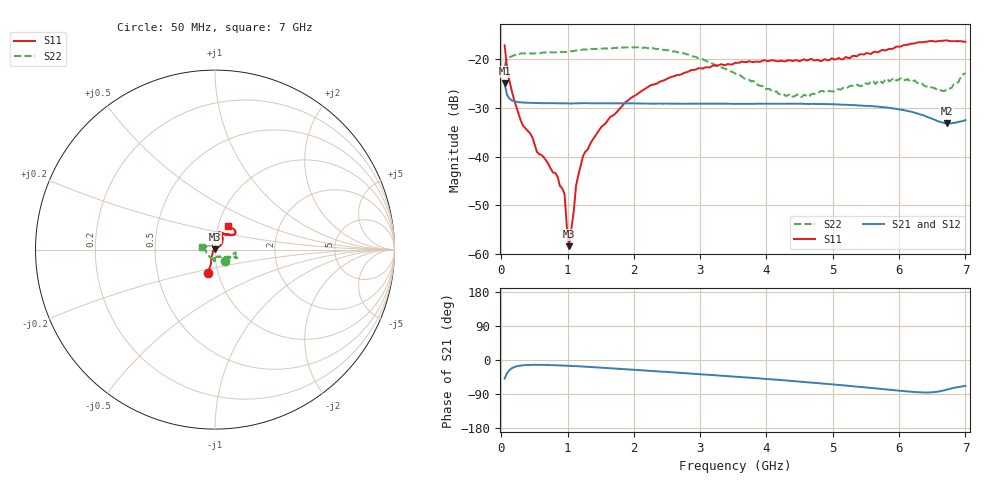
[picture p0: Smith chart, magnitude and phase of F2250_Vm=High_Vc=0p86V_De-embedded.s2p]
! Integrated Device Technology
! Corporate Headquarters
! 6024 Silver Creek Valley Road
! San Jose, CA 95138  USA
! Phone:  1-408-284-8200
! Toll Free:  1-800-223-1366
! Webpage:  http://www.idt.com/
! Timing and RF Division
! 515 Groton Road, Suite 102
! Westford, MA 01886-6024
! Device:  F2250
! Description: Voltage Variable RF Attenuator
! Frequency:  50.0 -  6000.00 MHz
! Package:  3x3 mm Thin QFN Plastic Package: 16 pin
! Ports:  2 RF, 3 DC
!  Pin  1  = GND
!  Pin  2  = NC
!  Pin  3  = RF1  = Port 1
!  Pin  4  = NC
!  Pin  5  = GND
!  Pin  6  = GND
!  Pin  7  = GND
!  Pin  8  = GND
!  Pin  9  = NC
!  Pin 10  = RF2  = Port 2
!  Pin 11  = NC
!  Pin 12  = GND
!  Pin 13  = GND
!  Pin 14  = VCNTRL
!  Pin 15  = VDD
!  Pin 16  = VMODE
! Vcntrl:  0.860 Volts
! Vmode:  +3.300 Volts
! Vdd:  +3.30  Volts
! Current:  1.310 mA
! Data:  The device was measured on a the F2250 evaluation board which has
!  individual transmission lines to the RF pins.  Data was collected
!  using a calibrated network analyzer.  The evaluation board was
!  de-embedded using a TRL calibration technique.
!  The reference plane is the edge of the package pin.
! Misc:  SN 10
!  Action Tracker AT0258
! Date Measured:  2014-11-26
! Date:  2015-10-15  MJV
! Note:
!  Integrated Device Technology supplies this data as a sample of measured
!  data at the package pin for this product.  Your particular data for this
!  product may vary.
!  Data was taken at 25 degrees C.
!  Integrated Device Technology reserves the right to change this data at anytime.
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# GHz S dB R 50
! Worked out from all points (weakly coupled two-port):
!   201 points, 50 MHz to 7 GHz, reference 50 ohm
!   highest |S21| = -24.91 dB at 50 MHz (marker M1); lowest = -33.2 dB at 6.722 GHz (marker M2)
!   lowest |S11| = -58.4 dB at 1.023 GHz (marker M3), VSWR 1.00, Z = 50 + j0.114 ohm
!   |S11| at or under -10 dB: start of sweep to end of sweep
!   |S22| runs from -27.8 to -17.6 dB; largest |S21 - S12| = 0.00016
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0.05  -17.16 -107.3  -24.91 -49.3  -24.92 -49.2  -21.40 -48.1
0.1195  -24.25 -110.0  -28.06 -27.1  -28.06 -27.1  -19.58 -13.9
0.29325  -32.59 -123.0  -28.86 -14.7  -28.84 -14.7  -18.84 -9.1
0.467  -35.97 -141.0  -28.97 -12.7  -28.98 -12.7  -18.85 -8.3
0.5365  -38.98 -148.4  -29.01 -12.7  -29.01 -12.7  -18.78 -9.4
0.84925  -44.11 172.2  -29.04 -14.1  -29.04 -14.1  -18.57 -13.6
0.9535  -47.62 175.2  -29.07 -14.8  -29.06 -14.8  -18.56 -14.7
0.98825  -54.28 169.2  -29.06 -15.0  -29.08 -15.0  -18.52 -15.0
1.023  -58.36 108.7  -29.08 -15.3  -29.09 -15.3  -18.42 -15.1
1.0925  -51.28 46.9  -29.07 -15.9  -29.06 -15.9  -18.34 -15.6
1.12725  -45.99 38.2  -29.05 -16.2  -29.05 -16.2  -18.23 -16.3
1.2315  -39.93 30.5  -29.03 -17.2  -29.02 -17.2  -18.03 -17.7
1.5095  -33.91 35.4  -29.05 -20.3  -29.04 -20.3  -17.86 -18.8
1.857  -29.01 36.3  -29.07 -24.2  -29.07 -24.2  -17.58 -20.3
2.37825  -24.74 44.7  -29.11 -30.2  -29.11 -30.2  -17.87 -21.3
3.525  -20.77 70.8  -29.17 -44.0  -29.17 -44.0  -22.93 -35.1
4.2895  -20.45 75.1  -29.15 -53.9  -29.15 -53.9  -27.55 -67.8
4.7065  -20.21 71.5  -29.17 -60.0  -29.20 -59.9  -27.07 -85.7
5.85325  -17.87 40.0  -30.00 -78.4  -30.00 -78.6  -24.55 -91.5
6.027  -17.42 38.4  -30.37 -81.3  -30.37 -81.4  -23.90 -93.6
6.722  -16.16 48.9  -33.19 -78.0  -33.20 -78.1  -26.03 -158.3
7  -16.43 62.0  -32.49 -68.2  -32.48 -68.4  -22.85 169.1
